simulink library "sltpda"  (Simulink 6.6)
InitFcn:
  | disp('Welcome to sLTPDA');
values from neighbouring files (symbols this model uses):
  hist = get(a, 'hist')    [string.m]    (also in display.m; save.m = a.hist; xml_read.m = xml_read_hist(ch))
  out = [t x]    [export.m]
  plist = [plist cellstr(p.key)]    [sltpda_control.m]
undefined symbols (not defined in the file or in its folder): ao, filter, foo_iir, Hanning, highpass, Kaiser, linear, param, pole, pzmodel

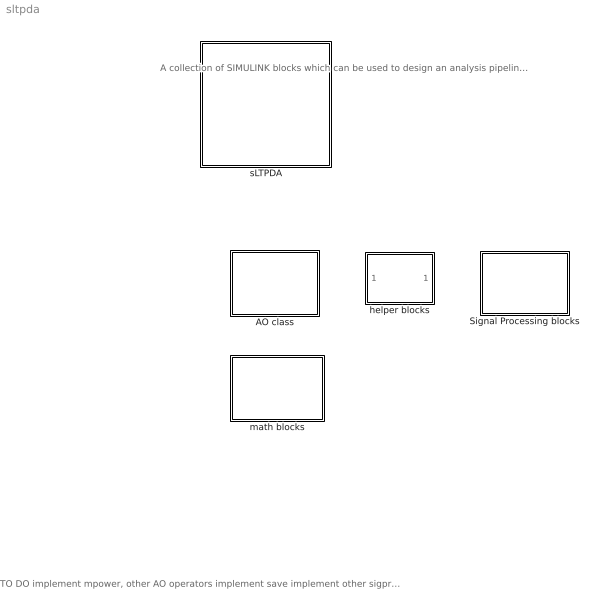
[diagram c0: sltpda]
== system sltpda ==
  note: A collection of SIMULINK blocks which can be used to design an analysis pipeline using LTPDA functions. The sLTPDA function set can be used to parse and run the model.
  note: TO DO implement mpower, other AO operators implement save implement other sigproc functions
  AO class : Subsystem
  Signal Processing blocks : Subsystem
  helper blocks : Subsystem
  math blocks : Subsystem
  sLTPDA : Subsystem

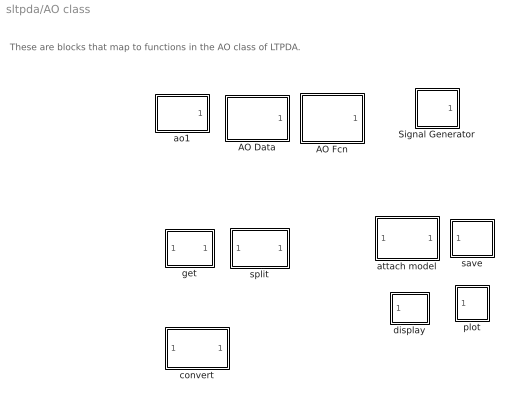
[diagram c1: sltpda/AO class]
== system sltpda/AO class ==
  note: These are blocks that map to functions in the AO class of LTPDA.
  AO Data : Subsystem  Tag=ao  mask(ao){vals=0}
      mask prompts: vals "data value(s)"
  AO Fcn : Subsystem  Tag=ao  mask(ao){fcn=0}
      mask prompts: fcn "Function"
  Signal Generator : Subsystem  Tag=ao  mask(ao){nsecs=1, fs=100, tsfcn=sin(2*pi*10*t)}
      mask prompts: nsecs "Num seconds"; fs "Sample rate"; tsfcn "Function y(t)"
  ao1 : Subsystem  Tag=ao  Description=Creates an Analysis object from a file.  mask(ao){fname=}
      mask prompts: fname "filename"
  attach model : Subsystem  Tag=attachdmdl
  convert : Subsystem  mask(convert){fcn=ao}
      mask prompts: fcn "convert to"
  display : Subsystem  Tag=display
  get : Subsystem  Tag=get  Description=Get the propery of an analysis object.  mask(get){param=hist}
      mask prompts: param "parameter"
  plot : Subsystem  Tag=plot  Description=Plot an analysis object.  mask(plot){xscale=linear, yscale=linear}
      mask prompts: xscale "x-scale"; yscale "y-scale"
  save : Subsystem  Tag=save  mask(save){fname=out.xml}
      mask prompts: fname "Filename"
  split : Subsystem  Tag=split  Description=Splits an AO into many sub-AOs.  mask(split){method=times, splits=0}
      mask prompts: method "splitting method"

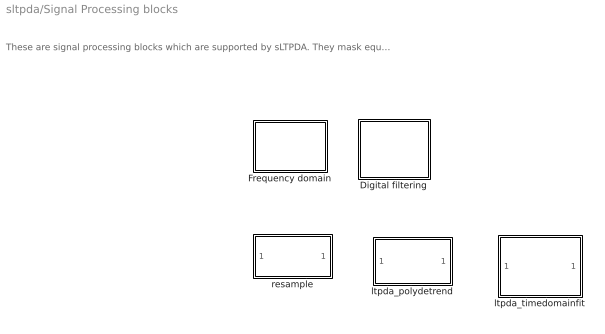
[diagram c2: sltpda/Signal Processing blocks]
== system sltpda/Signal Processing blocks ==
  note: These are signal processing blocks which are supported by sLTPDA. They mask equivalent functions which are in LTPDA.
  Digital filtering : Subsystem
  Frequency domain : Subsystem
  ltpda_polydetrend : Subsystem  Tag=ltpda_polydetrend  mask(ltpda_polydetrend){degree=1}
      mask prompts: degree "Degree of polynomial"
  ltpda_timedomainfit : Subsystem  Tag=ltpda_timedomainfit  Description=Performs a time-domain fit of the input AOs using ltpda_timedomainfit.
  resample : Subsystem  Tag=resample  mask(resample){fsout=0}
      mask prompts: fsout "Output sample rate"

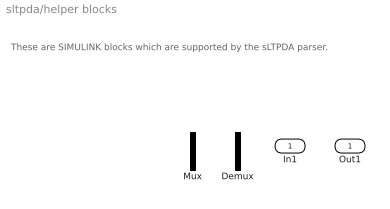
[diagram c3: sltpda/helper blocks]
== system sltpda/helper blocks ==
  note: These are SIMULINK blocks which are supported by the sLTPDA parser.
  In1 : Inport
  Demux : Demux  Outputs=2
  Mux : Mux  Inputs=2
  Out1 : Outport

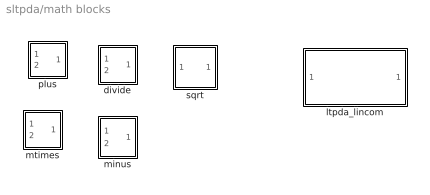
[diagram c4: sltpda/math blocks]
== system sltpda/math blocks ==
  divide : Subsystem  Tag=mrdivide
  ltpda_lincom : Subsystem  mask(ltpda_lincom){coeffs=0}
      mask prompts: coeffs "coefficients"
  minus : Subsystem  Tag=minus
  mtimes : Subsystem  Tag=mtimes
  plus : Subsystem  Tag=plus
  sqrt : Subsystem  Tag=sqrt

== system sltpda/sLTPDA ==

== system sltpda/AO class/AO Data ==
  Out1 : Outport

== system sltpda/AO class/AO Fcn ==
  Out1 : Outport

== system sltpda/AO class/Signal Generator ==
  Out1 : Outport

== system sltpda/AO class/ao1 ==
  out : Outport

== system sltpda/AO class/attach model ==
  In1 : Inport
  Out1 : Outport

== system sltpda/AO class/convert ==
  In1 : Inport
  Out1 : Outport

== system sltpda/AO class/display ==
  In1 : Inport

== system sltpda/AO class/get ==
  ao in : Inport
  property out : Outport

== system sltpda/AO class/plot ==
  ao in : Inport

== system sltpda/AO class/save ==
  In1 : Inport

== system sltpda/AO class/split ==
  In1 : Inport
  Out1 : Outport

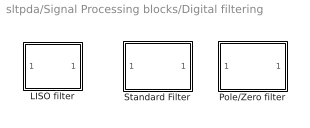
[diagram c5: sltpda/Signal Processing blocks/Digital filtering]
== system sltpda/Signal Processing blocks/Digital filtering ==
  LISO filter : Subsystem  Tag=filter  Description=Filter an AO.  mask(filter){fname=foo_iir.fil, method=filter}
      mask prompts: fname "filename"; method "filter method"
  Pole/Zero filter : Subsystem  mask(filter){method=filter, miirstr=pzmodel(plist([param('name', 'pzmodel') param('gain', [1]) param('poles', [ pole(plist([param('f', [1]) param('q', [0]) ]))]) param('zeros', []) ]))}
      mask prompts: method "filter method"; miirstr "constructor string"
      mask help: Filter using an IIR filter based on a pole/zero design. Use pzmodel_helper GUI to create the miir constructor string.
  Standard Filter : Subsystem  Tag=filter  Description=Apply a standard filter type to input AO.  mask(filter){method=filter, ftype=highpass, fgain=1, ffc=0.5, forder=1}
      mask prompts: ftype "filter type"; fgain "gain"; ffc "corner frequencie(s) [Hz]"; forder "filter order"

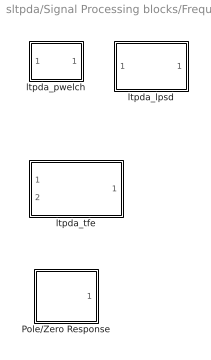
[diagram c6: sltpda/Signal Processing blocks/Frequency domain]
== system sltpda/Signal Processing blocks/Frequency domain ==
  Pole/Zero Response : Subsystem  mask(pzmresp){pzm=pzmodel(plist([param('name', 'pzmodel') param('gain', [1]) param('poles', [ pole(plist([param('f', [1]) param('q', [0]) ]))]) param('zeros', []) ])), f1=0.1, f2=100, nf=1000}
      mask prompts: pzm "pzmodel constructor"; f1 "start frequency"; f2 "stop frequency"; nf "num points"
  ltpda_lpsd : Subsystem  Tag=ltpda_psd  mask(ltpda_lpsd){Kdes=100, Kmin=1, Jdes=100, win=Kaiser, psll=100, olap=0}
      mask prompts: Kdes "Desired num averages"; Kmin "Minimum num averages"; Jdes "Number of spectral frequencies"; win "Window"; olap "Overlap"
  ltpda_pwelch : Subsystem  Tag=ltpda_pwelch  Description=Makes a spectral density estimate by calling ltpda_pwlech.  mask(ltpda_pwelch){win=Hanning, nfft=0, psll=0, nolap=0}
      mask prompts: win "Window"; nolap "Overlap (samples)"
  ltpda_tfe : Subsystem  Tag=ltpda_tfe  Description=Calls ltpda_tfe.  mask(ltpda_tfe){win=Hanning, nfft=, psll=, nolap=}
      mask prompts: win "Window"; nolap "Overlap (samples)"
      mask help: Computes a transfer function estimate given the input and output of the system. This calls ltpda_tfe() which in turn calls tfestimate().

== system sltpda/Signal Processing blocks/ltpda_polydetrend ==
  In1 : Inport
  Out1 : Outport

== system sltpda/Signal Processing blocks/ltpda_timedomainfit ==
  In1 : Inport
  Out1 : Outport

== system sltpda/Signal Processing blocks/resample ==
  In1 : Inport
  Out1 : Outport

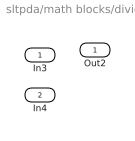
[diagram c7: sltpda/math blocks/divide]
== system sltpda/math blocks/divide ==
  In3 : Inport
  In4 : Inport  Port=2
  Out2 : Outport

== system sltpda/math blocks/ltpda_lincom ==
  In1 : Inport
  Out1 : Outport

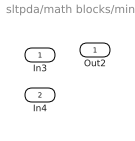
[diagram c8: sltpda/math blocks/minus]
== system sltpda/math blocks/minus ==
  In3 : Inport
  In4 : Inport  Port=2
  Out2 : Outport

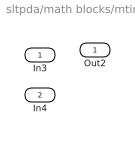
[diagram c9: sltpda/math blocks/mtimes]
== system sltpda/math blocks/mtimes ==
  In3 : Inport
  In4 : Inport  Port=2
  Out2 : Outport

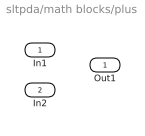
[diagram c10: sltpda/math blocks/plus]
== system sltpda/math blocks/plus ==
  In1 : Inport
  In2 : Inport  Port=2
  Out1 : Outport

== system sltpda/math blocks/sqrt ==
  In1 : Inport
  Out1 : Outport

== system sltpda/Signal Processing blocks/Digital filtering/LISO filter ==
  ao in : Inport
  property out : Outport

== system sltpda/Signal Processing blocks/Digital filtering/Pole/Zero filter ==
  In1 : Inport
  Out1 : Outport

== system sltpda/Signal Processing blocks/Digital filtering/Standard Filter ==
  In1 : Inport
  Out1 : Outport

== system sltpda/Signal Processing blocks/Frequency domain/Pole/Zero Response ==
  Out1 : Outport

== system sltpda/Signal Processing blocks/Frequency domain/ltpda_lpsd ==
  In1 : Inport
  Out1 : Outport

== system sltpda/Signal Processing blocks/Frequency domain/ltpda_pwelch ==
  In1 : Inport
  Out1 : Outport

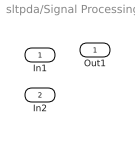
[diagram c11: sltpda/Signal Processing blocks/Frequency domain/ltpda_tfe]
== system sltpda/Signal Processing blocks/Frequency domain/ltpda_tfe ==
  In1 : Inport
  In2 : Inport  Port=2
  Out1 : Outport
